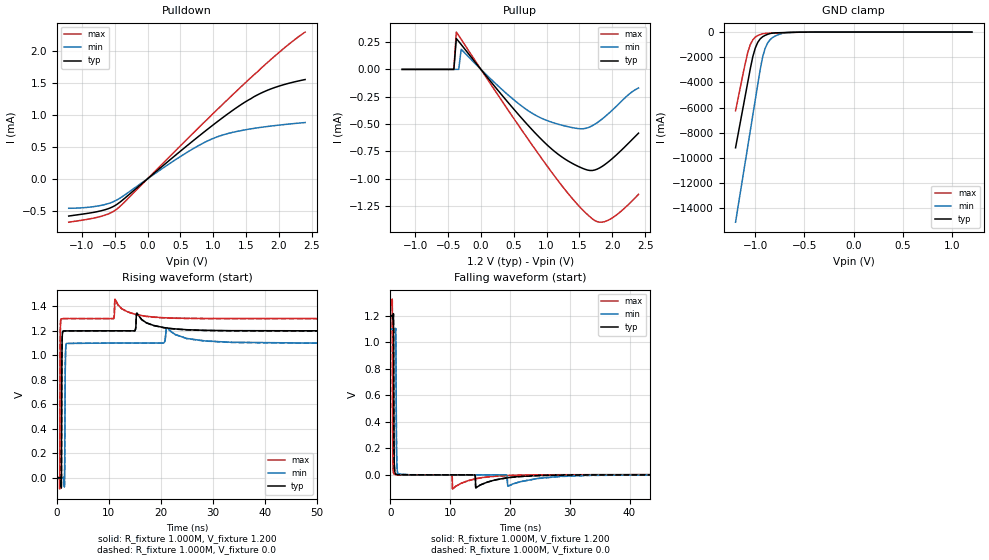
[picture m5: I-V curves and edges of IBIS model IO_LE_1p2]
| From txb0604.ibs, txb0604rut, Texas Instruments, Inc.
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|   Model IO_LE_1p2
[Model] IO_LE_1p2
Model_type 3-state
Polarity   Non-Inverting
Enable   Active-High
Vmeas =  0.600V
Cref =  15.000pF
Rref =  1.000M
Vref =  0.0V
C_comp   3.930pF   3.640pF   4.130pF
[Temperature Range]   27.000   0.125k   -40.000
[Voltage Range]   1.200V   1.100V   1.300V
[Pullup Reference]   1.200V   1.100V   1.300V
[Pulldown Reference]   0.0V   0.0V   0.0V
[POWER Clamp Reference]   1.200V   1.100V   1.300V
[GND Clamp Reference]   0.0V   0.0V   0.0V
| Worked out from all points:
|   slope of the pulldown table from 0 to 0.18 V, typ, clamps not added: 1.15 kohm
|   slope of the pullup table from 0 to 0.18 V, typ, clamps not added: 1.35 kohm
|   GND clamp passes 1 mA (typ) near -0.43 V on its own axis
|   rising waveform, R_fixture 1.000M, V_fixture 1.200: 20-80 % time 67.6ps typ, 92.1ps min, 50.3ps max; typ from 0.001 V to 1.2 V
|   rising waveform, R_fixture 1.000M, V_fixture 0.0: 20-80 % time 67.5ps typ, 91.8ps min, 50.1ps max; typ from 0 V to 1.2 V
|   falling waveform, R_fixture 1.000M, V_fixture 1.200: 20-80 % time 61.7ps typ, 88.1ps min, 52.6ps max; typ from 1.2 V to 0.001 V
|   falling waveform, R_fixture 1.000M, V_fixture 0.0: 20-80 % time 61.8ps typ, 88.5ps min, 52.7ps max; typ from 1.2 V to 0 V
[Pulldown]
|Voltage   I(typ)   I(min)   I(max)
-1.2V     -581.9uA   -460.3uA   -677.9uA
-719mV    -502.7uA   -417.8uA   -589.9uA
-571mV    -456.4uA   -378.3uA   -537.1uA
-460mV    -395.4uA   -327uA     -467.5uA
502mV     432.8uA    348.8uA    517uA
798mV     679.6uA    530.4uA    817.4uA
1.02V     858.4uA    639.3uA    1.04mA
1.205V    1.001mA    702.3uA    1.223mA
1.427V    1.161mA    752.3uA    1.44mA
1.723V    1.336mA    803.5uA    1.721mA
2.019V    1.454mA    840.8uA    1.989mA
2.4V      1.551mA    879.4uA    2.293mA
[Pullup]
|Voltage   I(typ)   I(min)   I(max)
-1.2V     175.5pA    1.627nA    829.1pA
-412mV    106.7nA    3.842nA    248.6nA
-375mV    282.5uA    43.21nA    341.9uA
-338mV    255.9uA    43.05nA    309.4uA
-301mV    228.2uA    184.3uA    275.8uA
328mV     -241.5uA   -188uA     -296.2uA
772mV     -547.7uA   -398.7uA   -685.7uA
1.216V    -795.1uA   -508.6uA   -1.052mA
1.66V     -926.1uA   -526.8uA   -1.35mA
1.771V    -913.4uA   -487.9uA   -1.395mA
1.919V    -857.3uA   -417.6uA   -1.387mA
2.4V      -583.9uA   -169.7uA   -1.144mA
[GND_clamp]
|Voltage   I(typ)   I(min)   I(max)
-1.2V     -9.186A    -15.09A    -6.25A
-1.075V   -3.941A    -9.027A    -1.583A
-1.025V   -1.957A    -6.601A    -615mA
-1V       -1.272A    -5.388A    -399.7mA
-975mV    -819.4mA   -4.175A    -276mA
-925mV    -369.8mA   -1.974A    -131.5mA
-900mV    -261mA     -1.3A      -105.2mA
-875mV    -181mA     -875mA     -93.58mA
-825mV    -80.65mA   -440mA     -80.5mA
-725mV    -43.5mA    -98.28mA   -56.44mA
-625mV    -20.69mA   -20.96mA   -26.75mA
1.2V      0A         0A         0A
[Ramp]
| variable   typ   min   max
dV/dt_r   0.719/66.589p   0.659/91.118p   0.779/51.681p
dV/dt_f   0.719/65.306p   0.659/89.413p   0.779/51.093p
R_load = 1.000M
[Rising Waveform]
R_fixture= 1.000M
V_fixture= 1.200
V_fixture_min= 1.100
V_fixture_max= 1.300
|time   V(typ)   V(min)   V(max)
0s        1.37mV     1.66mV     1.251mV
540ps     1.051mV    1.67mV     -90.93mV
620ps     860.3uV    1.651mV    1.025V
740ps     5.933mV    1.582mV    1.29V
850ps     -82.29mV   1.449mV    1.298V
1.13ns    1.195V     2.208mV    1.299V
1.47ns    1.199V     -41.69mV   1.299V
1.75ns    1.199V     1.087V     1.3V
11.2ns    1.2V       1.1V       1.459V
120ns     1.2V       1.1V       1.3V
[Rising Waveform]
R_fixture= 1.000M
V_fixture= 0.0
V_fixture_min= 0.0
V_fixture_max= 0.0
|time   V(typ)   V(min)   V(max)
0s        632nV      144.5uV    -1.372uV
540ps     -319.7uV   154.9uV    -92.21mV
620ps     -523.5uV   136.5uV    1.024V
740ps     4.499mV    67.44uV    1.29V
850ps     -83.72mV   -68.2uV    1.298V
1.13ns    1.195V     633.8uV    1.299V
1.47ns    1.198V     -43.38mV   1.299V
1.75ns    1.199V     1.087V     1.3V
11.2ns    1.2V       1.1V       1.459V
120ns     1.198V     1.098V     1.299V
[Falling Waveform]
R_fixture= 1.000M
V_fixture= 1.200
V_fixture_min= 1.100
V_fixture_max= 1.300
|time   V(typ)   V(min)   V(max)
0s        1.2V       1.1V       1.3V
330ps     1.197V     1.1V       1.303V
410ps     1.182V     1.101V     198.9mV
560ps     825.6mV    1.097V     10.92mV
670ps     79.51mV    1.087V     4.514mV
910ps     4.652mV    1.081V     2.397mV
1.03ns    3.04mV     233.2mV    1.901mV
1.25ns    2.138mV    10.73mV    1.258mV
10.41ns   25.13uV    41.07uV    -108mV
120ns     1.396mV    1.707mV    1.256mV
[Falling Waveform]
R_fixture= 1.000M
V_fixture= 0.0
V_fixture_min= 0.0
V_fixture_max= 0.0
|time   V(typ)   V(min)   V(max)
0s        1.198V     1.098V     1.299V
330ps     1.196V     1.098V     1.302V
410ps     1.18V      1.099V     198.5mV
560ps     824.2mV    1.096V     10.89mV
670ps     79.22mV    1.085V     4.487mV
910ps     4.624mV    1.079V     2.376mV
1.03ns    3.015mV    232.6mV    1.879mV
1.25ns    2.114mV    10.66mV    1.237mV
10.41ns   4.745uV    19.45uV    -108.1mV
120ns     27.53uV    191.6uV    4.169uV
